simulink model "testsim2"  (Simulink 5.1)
settings: Solver=ode23tb  StartTime=0.0  StopTime=1200  MaxStep=0.1  RelTol=1e-6
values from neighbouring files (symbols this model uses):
  c0 = [0 0 1]    [runcases.m]
  c1 = [0 1 1]    [runcases.m]
  f0 = [0 0 0]    [runcases.m]
  f1 = [0 1 2]    [runcases.m]
  l0 = [0 0 0]    [runcases.m]
  l1 = [0 0 1]    [runcases.m]
  t0 = [1 1 1]    [runcases.m]
  t1 = [1 0.95 0.95]    [runcases.m]
  tc = [0;140;0]    [runcases.m]
  tflt = [0;110;100]    [runcases.m]
  tl = [0;0;140]    [runcases.m]
  tt = [0;140;140]    [runcases.m]
undefined symbols (not defined in the file or in its folder): openloop, primarycontroller

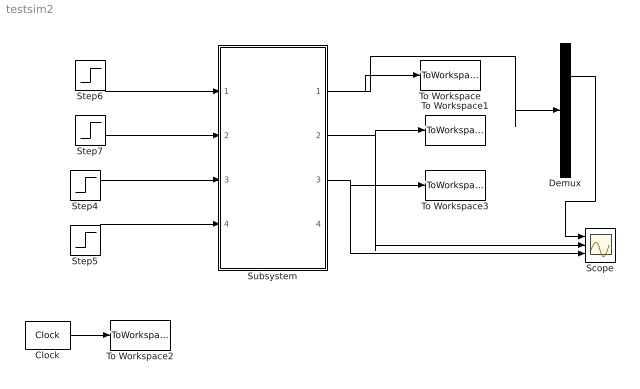
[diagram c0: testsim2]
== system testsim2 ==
  Clock : Clock
  Demux : Demux  Outputs=[3 2 3]
  Scope : Scope  NumInputPorts=3
  Step4 : Step  Time=tt  Before=t0  After=t1  SampleTime=0
  Step5 : Step  Time=tflt  Before=f0  After=f1  SampleTime=0
  Step6 : Step  Time=tc  Before=c0  After=c1  SampleTime=0
  Step7 : Step  Time=tl  Before=l0  After=l1  SampleTime=0
  Subsystem : Subsystem
  To Workspace : ToWorkspace  VariableName=V  SampleTime=-1  SaveFormat=Array
  To Workspace1 : ToWorkspace  VariableName=Efd  SampleTime=-1  SaveFormat=Array
  To Workspace2 : ToWorkspace  VariableName=t  SampleTime=-1  SaveFormat=Array
  To Workspace3 : ToWorkspace  VariableName=tappos  SampleTime=-1  SaveFormat=Array
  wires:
  Subsystem/1(V) -> To Workspace/1, Demux/1
  Clock/1 -> To Workspace2/1
  Subsystem/3(Tappos) -> To Workspace3/1, Scope/3
  Subsystem/2(Efd) -> To Workspace1/1, Scope/2
  Demux/1 -> Scope/1
  Step5/1 -> Subsystem/4(Faulted)
  Step7/1 -> Subsystem/2(LoadStep)
  Step4/1 -> Subsystem/3(TapVref)
  Step6/1 -> Subsystem/1(CapStep)

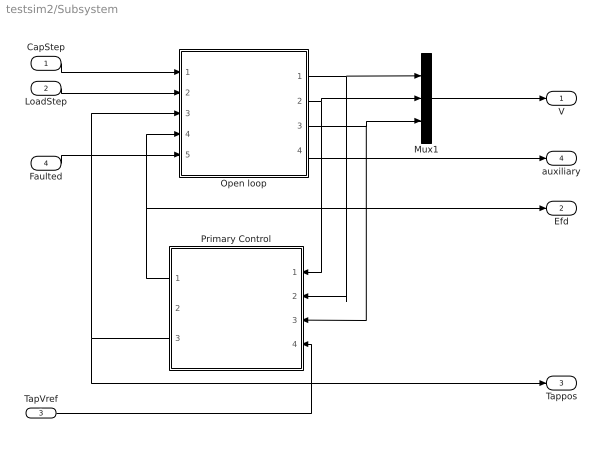
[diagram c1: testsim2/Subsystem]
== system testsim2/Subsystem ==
  CapStep : Inport
  LoadStep : Inport  Port=2
  TapVref : Inport  Port=3
  Faulted : Inport  Port=4
  Mux1 : Mux  Inputs=3
  Open loop : Subsystem
  Primary Control : Subsystem  Orientation=left
  V : Outport
  Efd : Outport  Port=2
  Tappos : Outport  Port=3
  auxiliary : Outport  Port=4
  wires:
  Open loop/1(Vload) -> Mux1/1, Primary Control/2(Vload)
  Open loop/2(Vgen) -> Primary Control/1(Vgen), Mux1/2
  Open loop/3(Vcap) -> Primary Control/3(Vcap), Mux1/3
  Primary Control/2(tappos) -> Open loop/3(TrStep), Tappos/1
  Primary Control/1("Efd ") -> Open loop/4(Efd), Efd/1
  CapStep/1 -> Open loop/1(CapStep)
  LoadStep/1 -> Open loop/2(LoadStep)
  Mux1/1 -> V/1
  Open loop/4("auxilliary ") -> auxiliary/1
  Faulted/1 -> Open loop/5(faulted)
  TapVref/1 -> Primary Control/4(TapVref)

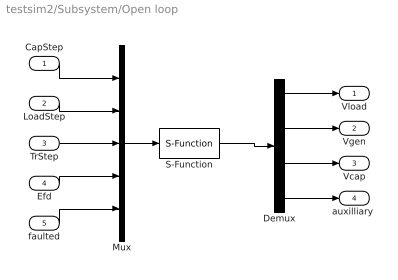
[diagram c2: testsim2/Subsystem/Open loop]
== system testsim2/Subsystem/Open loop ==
  CapStep : Inport
  LoadStep : Inport  Port=2
  TrStep : Inport  Port=3
  Efd : Inport  Port=4
  faulted : Inport  Port=5
  Demux : Demux  Outputs=[3 2 3 78]
  Mux : Mux  Inputs=[3 3 3 2 3]
  S-Function : S-Function  FunctionName=openloopd  Parameters=openloop.p,openloop.x0
  Vload : Outport
  Vgen : Outport  Port=2
  Vcap : Outport  Port=3
  "auxilliary " : Outport  Port=4
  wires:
  Mux/1 -> S-Function/1
  Demux/1 -> Vload/1
  Demux/2 -> Vgen/1
  S-Function/1 -> Demux/1
  CapStep/1 -> Mux/1
  LoadStep/1 -> Mux/2
  TrStep/1 -> Mux/3
  faulted/1 -> Mux/5
  Efd/1 -> Mux/4
  Demux/3 -> Vcap/1
  Demux/4 -> "auxilliary "/1

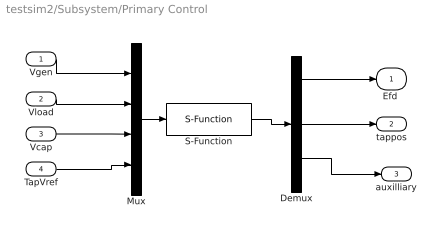
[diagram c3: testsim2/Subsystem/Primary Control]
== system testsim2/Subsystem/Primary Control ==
  Vgen : Inport
  Vload : Inport  Port=2
  Vcap : Inport  Port=3
  TapVref : Inport  Port=4
  Demux : Demux  Outputs=[2 3 14]
  Mux : Mux  Inputs=[2 3 3 3]
  S-Function : S-Function  FunctionName=primarycontrollerd  Parameters=primarycontroller.p,primarycontroller.x0
  "Efd " : Outport
  tappos : Outport  Port=2
  auxilliary : Outport  Port=3
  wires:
  Mux/1 -> S-Function/1
  S-Function/1 -> Demux/1
  Demux/1 -> "Efd "/1
  Demux/2 -> tappos/1
  Vgen/1 -> Mux/1
  Vload/1 -> Mux/2
  TapVref/1 -> Mux/4
  Vcap/1 -> Mux/3
  Demux/3 -> auxilliary/1
